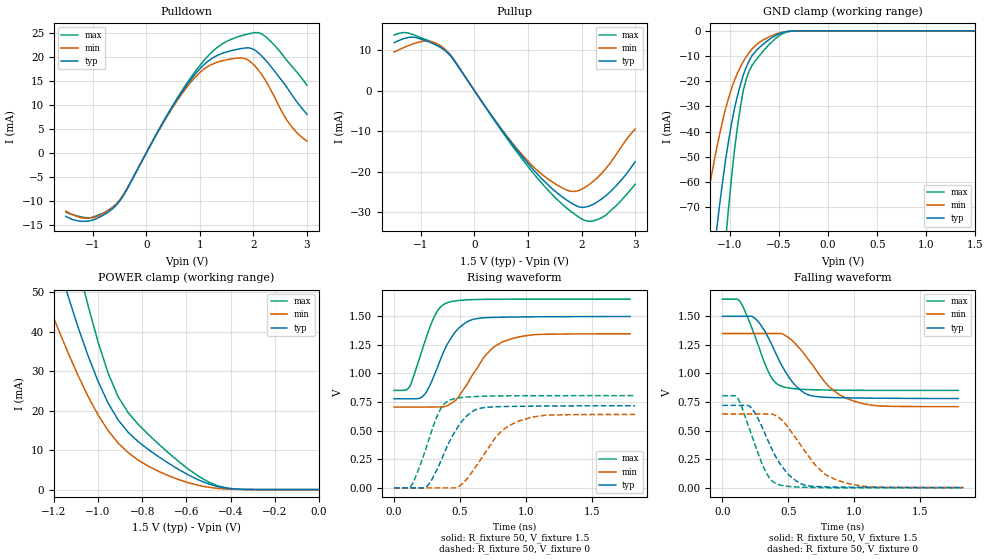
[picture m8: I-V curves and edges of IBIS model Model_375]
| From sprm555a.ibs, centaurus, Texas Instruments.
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| Model based on original model for BCSHTLTCSCDDVPBFZ_SSGFV
|   Sub model SR01_7MA_PADP_10PER_1P5
[model]   Model_375
|[Description]  [1.5V-3-STATE-X-FAST:7MA, IND, 10%]
|   Fast slew rate (SR[1:0] = "10"), 1.14 * RExt = 0.875 * Iout
|   (I[2:0] = "010"), 7mA nominal with Rext = 50R, ,Industrial
|   temperature range (-40C to 125C, 25C nominal),10% power supply
|   tolerance
|[Input Load]
|[Output Drive] FAST:7MA
|Voltage   1.5V
|Mode   3-STATE
Model_type   3-state
Polarity   Non-Inverting
Enable   Active-Low
Cref =  15pF
Rref =  100.0000M
Vref =  0V
Vmeas =  0.75
C_comp   1.865048p   1.676829p   1.989968p
[Temperature Range]   25   125   -40
[Voltage Range]   1.5   1.35   1.65
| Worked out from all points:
|   slope of the pulldown table from 0 to 0.225 V, typ, clamps not added: 48.9 ohm
|   slope of the pullup table from 0 to 0.225 V, typ, clamps not added: 51.5 ohm
|   GND clamp passes 1 mA (typ) near -0.49 V on its own axis
|   POWER clamp passes 1 mA (typ) near -0.47 V on its own axis
|   rising waveform, R_fixture 50, V_fixture 1.5: 20-80 % time 176ps typ, 233ps min, 144ps max; typ from 0.779 V to 1.5 V
|   rising waveform, R_fixture 50, V_fixture 0: 20-80 % time 190ps typ, 248ps min, 148ps max; typ from 0 V to 0.718 V
|   falling waveform, R_fixture 50, V_fixture 1.5: 20-80 % time 203ps typ, 274ps min, 159ps max; typ from 1.5 V to 0.781 V
|   falling waveform, R_fixture 50, V_fixture 0: 20-80 % time 197ps typ, 259ps min, 154ps max; typ from 0.721 V to 0.003 V
[POWER_clamp]
-1.5V     126mA      88.79mA    168.7mA
-1.242V   69.8mA     49.45mA    94.34mA
-1.136V   49.16mA    34.72mA    67.51mA
-1.061V   36.35mA    25.4mA     50.03mA
-1.045V   33.92mA    23.63mA    46.66mA
-954.5mV  21.93mA    14.95mA    29.5mA
-909.1mV  17.64mA    11.79mA    23.52mA
-863.6mV  14.51mA    9.351mA    19.47mA
-772.7mV  10.16mA    5.94mA     13.99mA
-590.9mV  3.705mA    1.741mA    5.166mA
-454.5mV  710.5uA    279.1uA    892.1uA
0V        1.424nA    14.34nA    3.127nA
[Pulldown]
-1.5V     -13.15mA   -12.08mA   -12.27mA
-1V       -13.92mA   -13.42mA   -13.31mA
-727.3mV  -12.4mA    -12.1mA    -12mA
-500mV    -10.04mA   -9.816mA   -9.874mA
272.7mV   5.543mA    5.395mA    5.589mA
681.8mV   12.92mA    12.52mA    13.17mA
1.045V    17.98mA    17.12mA    18.77mA
1.364V    20.43mA    18.95mA    22.21mA
1.818V    21.75mA    19.66mA    24.45mA
2.136V    20.34mA    16.6mA     24.8mA
2.636V    13.45mA    6.663mA    19.07mA
3V        8.041mA    2.506mA    14.06mA
[Pullup]
-1.5V     11.89mA    9.575mA    13.77mA
-1.182V   13.25mA    11.42mA    14.06mA
-954.5mV  12.56mA    12.25mA    12.88mA
-590.9mV  10.33mA    10.73mA    10.53mA
-409.1mV  7.967mA    8.059mA    8.155mA
909.1mV   -16.57mA   -16.13mA   -17.23mA
1.318V    -22.59mA   -21.31mA   -23.8mA
1.773V    -27.5mA    -24.81mA   -29.58mA
2.045V    -28.84mA   -24.06mA   -32.01mA
2.318V    -27.3mA    -21.21mA   -31.76mA
2.682V    -23mA      -15.08mA   -28.01mA
3V        -17.54mA   -9.488mA   -23.16mA
[GND_clamp]
-1.5V     -219.3mA   -131.6mA   -364.3mA
-1.288V   -134.4mA   -79.74mA   -225.6mA
-1.258V   -122.9mA   -72.77mA   -206.3mA
-1.136V   -79.27mA   -46.88mA   -132.4mA
-1.045V   -51.5mA    -31.06mA   -84.11mA
-1.015V   -44.02mA   -26.9mA    -70.91mA
-954.5mV  -31.01mA   -19.7mA    -47.55mA
-863.6mV  -17.48mA   -12.16mA   -23.55mA
-803mV    -11.81mA   -8.597mA   -15.85mA
-681.8mV  -5.986mA   -4.096mA   -9.026mA
-378.8mV  -126.2uA   -131.8uA   -179.7uA
1.5V      1.424nA    207.1nA    1.498nA
[Ramp]
dV/dt_f 0.43436406/0.20450156n 0.38757598/0.27691226n 0.48000839/0.1595904n
dV/dt_r 0.43418082/0.19204669n 0.38896257/0.25068645n 0.48490359/0.14810557n
R_load = 50
[Rising Waveform]
R_fixture = 50
V_fixture = 1.5
V_fixture_min = 1.35
V_fixture_max = 1.65
0s        778.7mV    706.2mV    852.4mV
116.5ps   778.7mV    706.2mV    881.8mV
222.3ps   806mV      706.2mV    1.241V
310.9ps   1.006V     707.5mV    1.511V
394.3ps   1.237V     714.3mV    1.614V
560.5ps   1.456V     921mV      1.644V
697.9ps   1.488V     1.166V     1.648V
830.6ps   1.492V     1.28V      1.649V
1.058ns   1.495V     1.339V     1.65V
1.787ns   1.498V     1.347V     1.65V
[Rising Waveform]
R_fixture = 50
V_fixture = 0
V_fixture_min = 0
V_fixture_max = 0
0s        0V         0V         0V
133.7ps   0V         0V         24.74mV
248.4ps   13.49mV    0V         368.8mV
347ps     216.2mV    0V         678.2mV
432.5ps   434.6mV    0V         771.4mV
503.8ps   568.2mV    23.4mV     788.8mV
608ps     678.3mV    168.2mV    798.2mV
785.5ps   709.6mV    464mV      803.6mV
939.8ps   713.1mV    581.7mV    805.1mV
1.825ns   718.1mV    641.7mV    806.2mV
[Falling Waveform]
R_fixture = 50
V_fixture = 1.5
V_fixture_min = 1.35
V_fixture_max = 1.65
0s        1.499V     1.349V     1.649V
127.6ps   1.499V     1.349V     1.637V
249.8ps   1.478V     1.349V     1.317V
361.7ps   1.281V     1.349V     983.7mV
449.3ps   1.071V     1.347V     887.6mV
535.3ps   918mV      1.281V     867.2mV
641.7ps   817.3mV    1.137V     858.9mV
805.8ps   790.2mV    886.6mV    854.5mV
966.5ps   785.9mV    770.2mV    852.6mV
1.787ns   780.9mV    709.9mV    851.4mV
[Falling Waveform]
R_fixture = 50
V_fixture = 0
V_fixture_min = 0
V_fixture_max = 0
0s        720.6mV    645.1mV    805.3mV
112.1ps   720.6mV    645.1mV    793.3mV
214.1ps   705.8mV    645.1mV    486.6mV
318.4ps   486.3mV    645.1mV    164.2mV
411.4ps   257.6mV    627.5mV    34.3mV
600.2ps   33.21mV    361.8mV    5.71mV
769.8ps   8.934mV    125.4mV    2.056mV
885.7ps   6.65mV     60.47mV    0V
1.09ns    4.901mV    10.47mV    0V
1.825ns   2.738mV    3.218mV    0V
